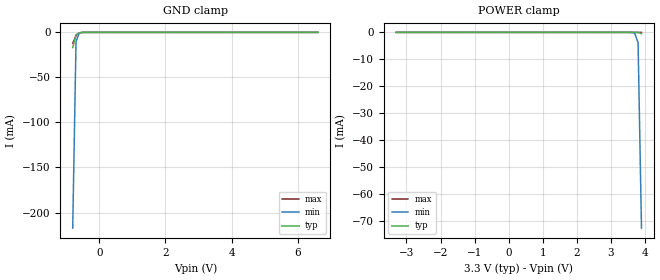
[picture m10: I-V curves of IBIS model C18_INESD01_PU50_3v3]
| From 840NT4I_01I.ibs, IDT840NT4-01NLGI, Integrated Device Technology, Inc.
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| 4.00000e+00   -2.70773e-03   -1.00314e+00   -1.11726e-04
| 4.10000e+00   -1.68690e-02   -2.32450e+00   -1.12643e-03
| 4.20000e+00   -4.41714e-01   -3.64703e+00   -5.94022e-03
| 4.30000e+00   -2.03108e+00   -4.97033e+00   -1.62279e-02
| 4.40000e+00   -3.62164e+00   -6.29417e+00   -7.71670e-02
| 4.50000e+00   -5.21297e+00   -7.61836e+00   -1.59470e+00
| 4.60000e+00   -6.80479e+00   -8.94280e+00   -3.63023e+00
| 4.70000e+00   -8.39688e+00   -1.02674e+01   -5.66630e+00
| 4.80000e+00   -9.98912e+00   -1.15920e+01   -7.70260e+00
| 4.90000e+00   -1.15814e+01   -1.29167e+01   -9.73893e+00
| 5.00000e+00   -1.31736e+01   -1.42413e+01   -1.17752e+01
| 5.10000e+00   -1.47658e+01   -1.55659e+01   -1.38112e+01
| 5.20000e+00   -1.63577e+01   -1.68904e+01   -1.58470e+01
| 5.30000e+00   -1.79495e+01   -1.82148e+01   -1.78825e+01
| 5.40000e+00   -1.95411e+01   -1.95390e+01   -1.99177e+01
| 5.50000e+00   -2.11325e+01   -2.08630e+01   -2.19525e+01
| 5.60000e+00   -2.27236e+01   -2.21870e+01   -2.39869e+01
| 5.70000e+00   -2.43145e+01   -2.35107e+01   -2.60210e+01
| 5.80000e+00   -2.59051e+01   -2.48343e+01   -2.80547e+01
| 5.90000e+00   -2.74954e+01   -2.61577e+01   -3.00881e+01
| 6.00000e+00   -2.90855e+01   -2.74809e+01   -3.21210e+01
| 6.10000e+00   -3.06753e+01   -2.88039e+01   -3.41536e+01
| 6.20000e+00   -3.22649e+01   -3.01267e+01   -3.61858e+01
| 6.30000e+00   -3.38541e+01   -3.14494e+01   -3.82177e+01
| 6.40000e+00   -3.54432e+01   -3.27718e+01   -4.02492e+01
| 6.50000e+00   -3.70319e+01   -3.40941e+01   -4.22803e+01
| 6.60000e+00   -3.86204e+01   -3.54162e+01   -4.43111e+01
[Model] C18_INESD01_PU50_3v3
Model_type   Input
Polarity   Non-Inverting
Vinl = 0.8V
Vinh = 2.0V
|   typ   min   max
C_comp   2pF   1.5pF   2.5pF
|   typ   min   max
[Voltage range]   3.3V   3.135V   3.465V
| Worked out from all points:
|   GND clamp passes 1 mA (typ) near -0.62 V on its own axis
[GND_clamp]
|Voltage   I (typ)   I (min)   I (max)
|Note, modeling breaks down at 250mA and above.  This is well beyond the functional   |
|operating range of the device.  Should this scenario occur, catastrophic failure and   |
|possible damage to the device and/or board is of higher concern than the I-V curve   |
|behavior.  The IBIS checker will flag currents in excess of 10A with warnings.  Lines   |
|with currents in excess of 0.35 A have been commented out.  The points still remain|
|available to the user if the user desires to use them.   |
|-3.30000e+00   -3.86204e+01   -3.32347e+01   -4.76611e+01
|-3.20000e+00   -3.70319e+01   -3.19123e+01   -4.56309e+01
|-3.10000e+00   -3.54431e+01   -3.05897e+01   -4.36003e+01
|-3.00000e+00   -3.38541e+01   -2.92669e+01   -4.15694e+01
|-2.90000e+00   -3.22648e+01   -2.79439e+01   -3.95382e+01
|-2.80000e+00   -3.06753e+01   -2.66208e+01   -3.75066e+01
|-2.70000e+00   -2.90855e+01   -2.52975e+01   -3.54746e+01
|-2.60000e+00   -2.74954e+01   -2.39740e+01   -3.34423e+01
|-2.50000e+00   -2.59051e+01   -2.26503e+01   -3.14095e+01
|-2.40000e+00   -2.43144e+01   -2.13264e+01   -2.93764e+01
|-2.30000e+00   -2.27236e+01   -2.00024e+01   -2.73430e+01
|-2.20000e+00   -2.11325e+01   -1.86782e+01   -2.53091e+01
|-2.10000e+00   -1.95411e+01   -1.73539e+01   -2.32749e+01
|-2.00000e+00   -1.79495e+01   -1.60295e+01   -2.12403e+01
|-1.90000e+00   -1.63577e+01   -1.47050e+01   -1.92054e+01
|-1.80000e+00   -1.47657e+01   -1.33803e+01   -1.71701e+01
|-1.70000e+00   -1.31736e+01   -1.20557e+01   -1.51345e+01
|-1.60000e+00   -1.15814e+01   -1.07310e+01   -1.30986e+01
|-1.50000e+00   -9.98911e+00   -9.40638e+00   -1.10625e+01
|-1.40000e+00   -8.39687e+00   -8.08189e+00   -9.02621e+00
|-1.30000e+00   -6.80478e+00   -6.75759e+00   -6.98987e+00
|-1.20000e+00   -5.21296e+00   -5.43362e+00   -4.95363e+00
|-1.10000e+00   -3.62163e+00   -4.11011e+00   -2.91770e+00
|-1.00000e+00   -2.03107e+00   -2.78727e+00   -8.82452e-01
|-9.00000e-01   -4.41704e-01   -1.46544e+00   -3.27936e-02
-800mV    -16.86mA   -217.3mA   -11.96mA
-700mV    -2.699mA   -10.28mA   -3.622mA
-600mV    -444.5uA   -692.6uA   -517uA
-400mV    -3.746uA   -7.6uA     -1.617uA
6.6V      278.6pA    1.056nA    218.7pA
[Power_clamp]
|Voltage   I (typ)   I (min)   I (max)
|Note, modeling breaks down at 250mA and above.  This is well beyond the functional   |
|operating range of the device.  Should this scenario occur, catastrophic failure and   |
|possible damage to the device and/or board is of higher concern than the I-V curve   |
|behavior.  The IBIS checker will flag currents in excess of 10A with warnings.  Lines   |
|with currents in excess of 0.35 A have been commented out.  The points still remain|
|available to the user if the user desires to use them.   |
-3.3V     278.6pA    998.4pA    224.3pA
3.5V      -10.53nA   -3.884uA   -6.094pA
3.7V      -3.746uA   -293.6uA   -3.16nA
3.8V      -47.41uA   -3.819mA   -176.4nA
3.9V      -444.5uA   -72.72mA   -5.07uA
